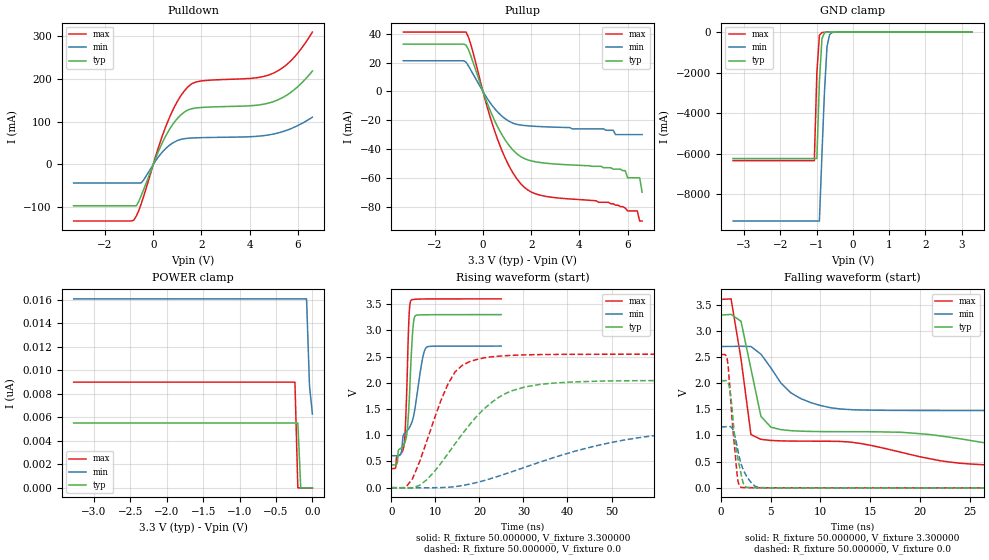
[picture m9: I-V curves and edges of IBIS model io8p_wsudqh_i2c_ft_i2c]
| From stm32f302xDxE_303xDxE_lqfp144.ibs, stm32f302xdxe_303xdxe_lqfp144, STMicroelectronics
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|   Model io8p_wsudqh_i2c_ft_i2c
[Model]  io8p_wsudqh_i2c_ft_i2c
Model_type I/O
Polarity   Non-Inverting
Enable   Active-Low
Vinl =   0.990000V
Vinh =   2.310000V
Vmeas =  1.650000V
Cref =   30.000000pF
Rref =   100.000000M
Vref =   0.0V
C_comp   0.0F   0.0F   0.0F
[Temperature Range]   25.000000   0.140000k   -40.000000
[Pullup Reference]   3.300000V   2.700000V   3.600000V
[Pulldown Reference]   0.0V   0.0V   0.0V
[POWER Clamp Reference]   3.300000V   2.700000V   3.600000V
[GND Clamp Reference]   0.0V   0.0V   0.0V
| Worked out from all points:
|   slope of the pulldown table from 0 to 0.495 V, typ, clamps not added: 7.75 ohm
|   slope of the pullup table from 0 to 0.495 V, typ, clamps not added: 23.9 ohm
|   GND clamp passes 1 mA (typ) near -0.61 V on its own axis
|   rising waveform, R_fixture 50.000000, V_fixture 3.300000: 20-80 % time 1.17ns typ, 3.82ns min, 775ps max; typ from 0.435 V to 3.3 V
|   rising waveform, R_fixture 50.000000, V_fixture 0.0: 20-80 % time 12.2ns typ, 29.8ns min, 6.8ns max; typ from 0 V to 2.04 V
|   falling waveform, R_fixture 50.000000, V_fixture 3.300000: 20-80 % time 18.9ns typ, 55.7ns min, 1.48ns max; typ from 3.3 V to 0.435 V
|   falling waveform, R_fixture 50.000000, V_fixture 0.0: 20-80 % time 807ps typ, 1.07ns min, 653ps max; typ from 2.04 V to 0 V
[Pulldown]
|Voltage   I(typ)   I(min)   I(max)
-3.3V     -96.33mA   -43.01mA   -131.7mA
-800mV    -96.33mA   -43.01mA   -129.4mA
-700mV    -96.33mA   -43.01mA   -120mA
-500mV    -72.9mA    -43.01mA   -92.16mA
200mV     28.44mA    16.57mA    37.01mA
600mV     74.69mA    41.37mA    99.56mA
1V        107.1mA    55.62mA    146.8mA
1.4V      125.8mA    60.81mA    178.5mA
1.9V      132.3mA    62.32mA    193.7mA
5V        146.7mA    71.07mA    213.2mA
5.8V      172.1mA    85.55mA    247mA
6.6V      217.6mA    110.1mA    308.5mA
[Pullup]
|Voltage   I(typ)   I(min)   I(max)
-3.3V     32.83mA    21.29mA    41.22mA
-700mV    32.15mA    20.31mA    41.22mA
200mV     -9.092mA   -5.447mA   -12.2mA
700mV     -27.48mA   -15.83mA   -37.39mA
1.2V      -39.86mA   -21.71mA   -55.32mA
1.8V      -47.22mA   -23.81mA   -67.73mA
5.7V      -54mA      -30mA      -80mA
5.9V      -55mA      -30mA      -81mA
6V        -60mA      -30mA      -83mA
6.4V      -60mA      -30mA      -83mA
6.5V      -60mA      -30mA      -90mA
6.6V      -70mA      -30mA      -90mA
[GND_clamp]
|Voltage   I(typ)   I(min)   I(max)
-3.3V     -6.241A    -9.325A    -6.345A
-1.06V    -6.241A    -9.325A    -6.345A
-990mV    -6.241A    -9.325A    -2.007A
-920mV    -2.435A    -9.325A    -157.2mA
-850mV    -331.1mA   -6.034A    -23.1mA
-780mV    -36.12mA   -2.918A    -12.65mA
-710mV    -6.437mA   -709.1mA   -7.385mA
-640mV    -1.621mA   -128.1mA   -3.348mA
-570mV    -372.4uA   -25.26mA   -954.9uA
3.28V     0A         5.405nA    0A
[POWER_clamp]
|Voltage   I(typ)   I(min)   I(max)
-3.28V    5.515nA    16.06nA    8.985nA
-240mV    5.515nA    16.06nA    8.985nA
-200mV    5.515nA    16.06nA    0A
-160mV    0A         16.06nA    0A
-80mV     0A         16.06nA    0A
-40mV     0A         8.703nA    0A
0V        0A         6.282nA    0A
[Ramp]
| variable   typ   min   max
dV/dt_r  1.22640/12.15891n   0.69888/29.73201n   1.52640/6.74730n
dV/dt_f  1.71911/18.80212n   1.25368/55.58701n   1.94084/1.26084n
R_load = 50.000000
[Rising Waveform]
R_fixture= 50.000000
V_fixture= 3.300000
V_fixture_min= 2.700000
V_fixture_max= 3.600000
|time   V(typ)   V(min)   V(max)
0s        434.9mV    609.3mV    365.2mV
2.102ns   748.1mV    638.4mV    642.5mV
2.903ns   832.1mV    1.031V     825.6mV
3.253ns   913.8mV    1.059V     1.316V
3.654ns   1.142V     1.093V     2.348V
4.054ns   1.674V     1.141V     3.343V
4.404ns   2.34V      1.197V     3.566V
5.205ns   3.241V     1.437V     3.591V
7.958ns   3.297V     2.677V     3.598V
24.92ns   3.3V       2.7V       3.6V
[Rising Waveform]
R_fixture= 50.000000
V_fixture= 0.0
V_fixture_min= 0.0
V_fixture_max= 0.0
|time   V(typ)   V(min)   V(max)
0s        1.147nV    13.92nV    972.5pV
3.203ns   -1.361mV   -685uV     561.8uV
4.805ns   -1.498mV   -966.5uV   172.7mV
11.21ns   461.7mV    1.512mV    1.655V
14.41ns   831.5mV    18.62mV    2.203V
20.82ns   1.486V     130.1mV    2.472V
28.83ns   1.885V     346.2mV    2.529V
57.66ns   2.041V     969.7mV    2.544V
99.3ns    2.044V     1.15V      2.544V
797.6ns   2.044V     1.165V     2.544V
[Falling Waveform]
R_fixture= 50.000000
V_fixture= 3.300000
V_fixture_min= 2.700000
V_fixture_max= 3.600000
|time   V(typ)   V(min)   V(max)
0s        3.3V       2.7V       3.6V
1.001ns   3.313V     2.702V     3.61V
2.002ns   3.183V     2.704V     2.462V
3.003ns   2.272V     2.7V       1.017V
4.004ns   1.366V     2.554V     926.9mV
5.005ns   1.159V     2.293V     905mV
11.01ns   1.074V     1.531V     889.7mV
28.03ns   811.9mV    1.475V     426.5mV
108.1ns   437.9mV    666.4mV    365.5mV
498.5ns   434.9mV    609.3mV    365.2mV
[Falling Waveform]
R_fixture= 50.000000
V_fixture= 0.0
V_fixture_min= 0.0
V_fixture_max= 0.0
|time   V(typ)   V(min)   V(max)
0s        2.044V     1.165V     2.544V
600.6ps   2.036V     1.171V     2.476V
700.7ps   2.009V     1.173V     2.348V
1.001ns   1.709V     1.161V     1.574V
1.301ns   1.086V     1.051V     885.7mV
1.602ns   650.7mV    799.4mV    268.9mV
2.002ns   268.2mV    463.9mV    11.3mV
2.402ns   29.04mV    278.3mV    4.977mV
3.904ns   2.449mV    6.683mV    1.925mV
49.85ns   1.147nV    13.92nV    972.5pV
